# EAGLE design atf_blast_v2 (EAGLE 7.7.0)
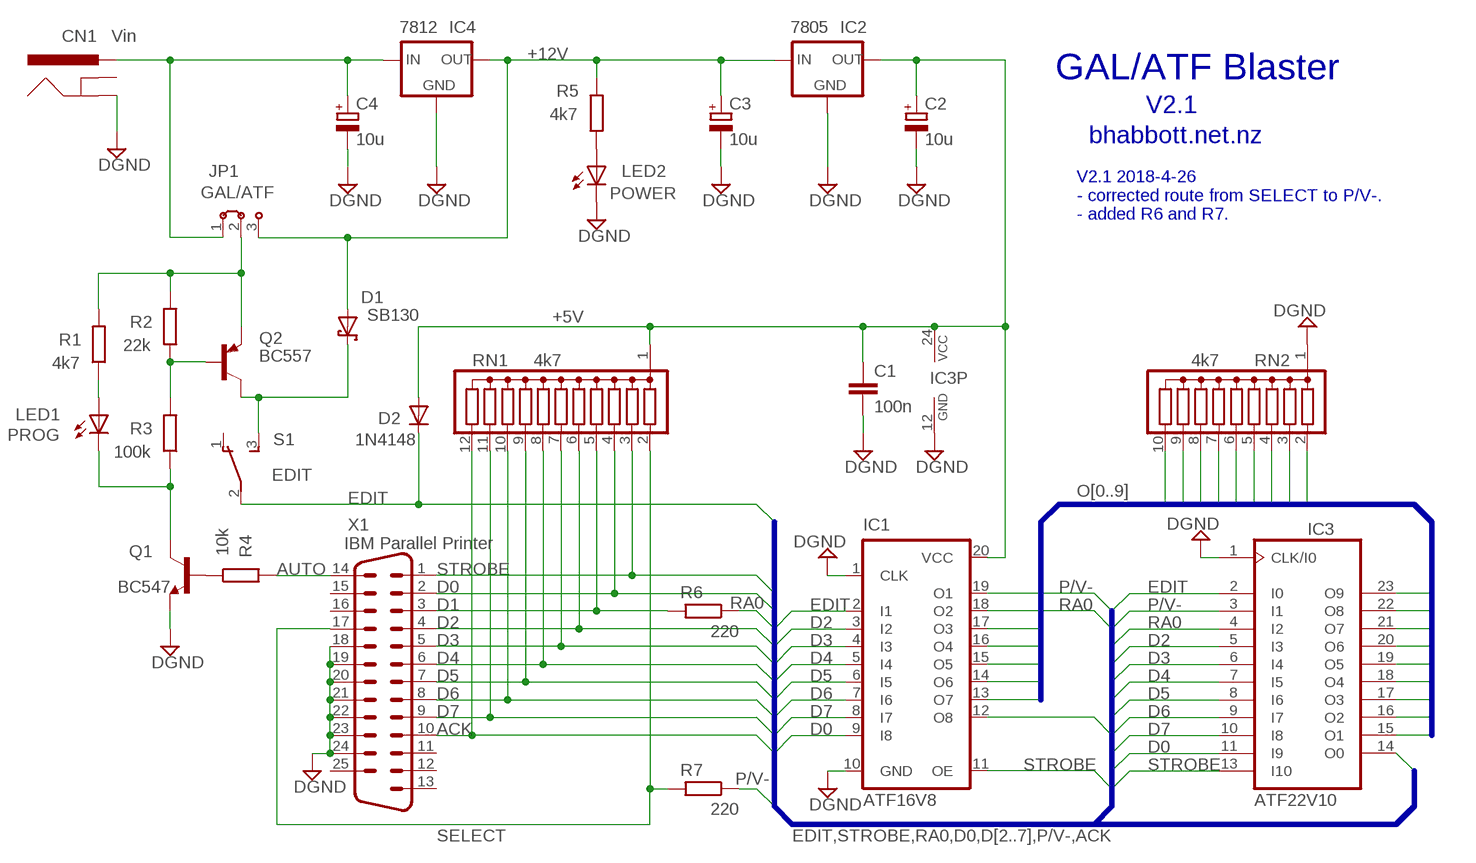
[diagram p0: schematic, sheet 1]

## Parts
C1  100n  C-EU025-024X044  [C025-024X044]
C2  10u  CPOL-EUE2.5-5  [E2,5-5]
C3  10u  CPOL-EUE2.5-5  [E2,5-5]
C4  10u  CPOL-EUE2.5-5  [E2,5-5]
CN1  Vin  POWER_JACKSLT  [POWER_JACK_SLOT]
D1  SB130  SCHOTTKY-DIODEDO35-7  [DO35-7]
D2  1N4148  1N4148DO35-7  [DO35-7]
IC1  ATF16V8  ATF16V8BP3  [DIL20]
IC2  7805  78XXLNV  [78XXL_GND]
IC3  ATF22V10  22V10  [DIL24-3]
IC4  7812  78XXLNV  [78XXL_GND]
JP1  GAL/ATF  JP2N  [0256]
LED1  PROG  LED5MM  [LED5MM]
LED2  POWER  LED5MM  [LED5MM]
Q1  BC547  [TO92]
Q2  BC557  [TO92]
R1  4k7  R-EU_0204/7  [0204/7]
R2  22k  R-EU_0204/7  [0204/7]
R3  100k  R-EU_0204/7  [0204/7]
R4  10k  R-EU_0204/7  [0204/7]
R5  4k7  R-EU_0204/7  [0204/7]
R6  220  R-EU_0204/7  [0204/7]
R7  220  R-EU_0204/7  [0204/7]
RN1  4k7  G11R  [SIL12]
RN2  4k7  G09R  [SIL10]
S1  EDIT  TL36PO  [TL3XPO]
X1  IBM Parallel Printer  M25HP  [M25HP]

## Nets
+5V: C1.1 C2.+ D2.A IC1.20(VCC) IC2.OUT IC3.24(VCC) RN1.1
+12V: C3.+ D1.A IC2.IN IC4.OUT JP1.3 R5.2
ACK: IC1.12(O8) IC3.14(O0) RN1.12 X1.10
AUTO: R4.2 X1.14
CN1: C4.+ CN1.PWR IC4.IN JP1.1
D0: IC1.9(I8) IC3.11(I9) RN1.4 X1.2
D1: R6.2 RN1.5 X1.3
D2: IC1.3(I2) IC3.5(I3) RN1.6 X1.4
D3: IC1.4(I3) IC3.6(I4) RN1.7 X1.5
D4: IC1.5(I4) IC3.7(I5) RN1.8 X1.6
D5: IC1.6(I5) IC3.8(I6) RN1.9 X1.7
D6: IC1.7(I6) IC3.9(I7) RN1.10 X1.8
D7: IC1.8(I7) IC3.10(I8) RN1.11 X1.9
DGND: C1.2 C2.- C3.- C4.- CN1.GND@2(GND) IC1.1(CLK) IC1.10(GND) IC2.GND IC3.1(CLK/I0) IC3.12(GND) IC4.GND LED2.K(C) Q1.1(E) RN2.1 X1.18 X1.19 X1.20 X1.21 X1.22 X1.23 X1.24
EDIT: D2.C IC1.2(I1) IC3.2(I0) S1.2(P)
N$1: D1.C Q2.3(C) S1.3(S)
N$2: Q2.2(B) R2.1 R3.2
N$3: LED1.K(C) Q1.3(C) R3.1
N$4: Q1.2(B) R4.1
N$6: LED1.A R1.1
N$7: JP1.2 Q2.1(E) R1.2 R2.2
N$22: LED2.A R5.1
O1: IC1.13(O7) IC3.15(O1) RN2.2
O2: IC1.14(O6) IC3.16(O2) RN2.3
O3: IC1.15(O5) IC3.17(O3) RN2.4
O4: IC1.16(O4) IC3.18(O4) RN2.5
O5: IC1.17(O3) IC3.19(O5) RN2.6
O6: IC3.20(O6) RN2.7
O7: IC3.21(O7) RN2.8
O8: IC3.22(O8) RN2.9
O9: IC3.23(O9) RN2.10
P/V-: IC1.19(O1) IC3.3(I1) R7.1
RA0: IC1.18(O2) IC3.4(I2) R6.1
SELECT: R7.2 RN1.2 X1.17
STROBE: IC1.11(OE) IC3.13(I10) RN1.3 X1.1
Unconnected: CN1.GND@1(GNDBREAK) S1.1(O) X1.11 X1.12 X1.13 X1.15 X1.16 X1.25 X1.G1 X1.G2

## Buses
EDIT,STROBE,RA0,D0,D[2..7],P/V-,ACK
O[0..9]

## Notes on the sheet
- GAL/ATF Blaster
- V2.1
- bhabbott.net.nz
- V2.1 2018-4-26 
  - corrected route from SELECT to P/V-. 
  - added R6 and R7.

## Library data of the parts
C1 = rcl:C-EU: CAPACITOR, European symbol
C2-C4 = rcl:CPOL-EU: POLARIZED CAPACITOR, European symbol
CN1 = SparkFun-Connectors:POWER_JACK: Power Jack This is the standard 5.5mm barrel jack for power. The PTH is the most common, proven, reliable, footprint. The Slot footprint only works if the mill layer is transmitted to the PCB fab house so be warned. Mating wall wart : TOL-00298 (and others); PROD_ID: PRT-00119
D1 = diode:SCHOTTKY-DIODE: Schottky Diode
D2 = diode:1N4148: DIODE
IC1 = atmel:ATF16V8B: High perfomance CMOS (electrically erasable) programmable logic device (PLD) ABLE-Atmel-ABEL - P18V8R, P16V8C, P16V8AS, P17V8 COPL Atmel-WinCUPL - G16V8MS, G16V8MA, G16V8AS, G16V8 LOG/IC - GAL16V8_R, GAL16V8_G7, GAL16V8_C), GAL16V8 Tango-PLD - G16V8R, G16V8C, G16V8AS, G16V8 Source: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; MPN: ATF16V8CZ-15PU; OC_FARNELL: 1551768; OC_NEWARK: 94M6254
IC2 IC4 = v-reg:78XXL: VOLTAGE REGULATOR
IC3 = pal:22V10: PAL; MPN: GAL22V10D-7LPN; OC_FARNELL: 1571925; OC_NEWARK: 97M0480
JP1 = jumper:JP2N: JUMPER 3 pin 0.1 inch
LED1 LED2 = led:LED: LED
Q1 = transistor-npn:BC547*: NPN Transistor
Q2 = transistor-pnp:BC557: PNP Transistor
R1-R7 = rcl:R-EU_: RESISTOR, European symbol
RN1 = resistor-sil:G11R: SIL RESISTOR; OC_FARNELL: unknown; OC_NEWARK: unknown
RN2 = resistor-sil:G09R: SIL RESISTOR
S1 = switch:TL36PO: TINY SWITCH ON - ON Source: http://www2.produktinfo.conrad.com/datenblaetter/700000-724999/705152-da-01-de-Subminiaturschalter_TL_36YO.pdf
X1 = con-subd:M25HP: SUB-D; OC_FARNELL: unknown; OC_NEWARK: unknown

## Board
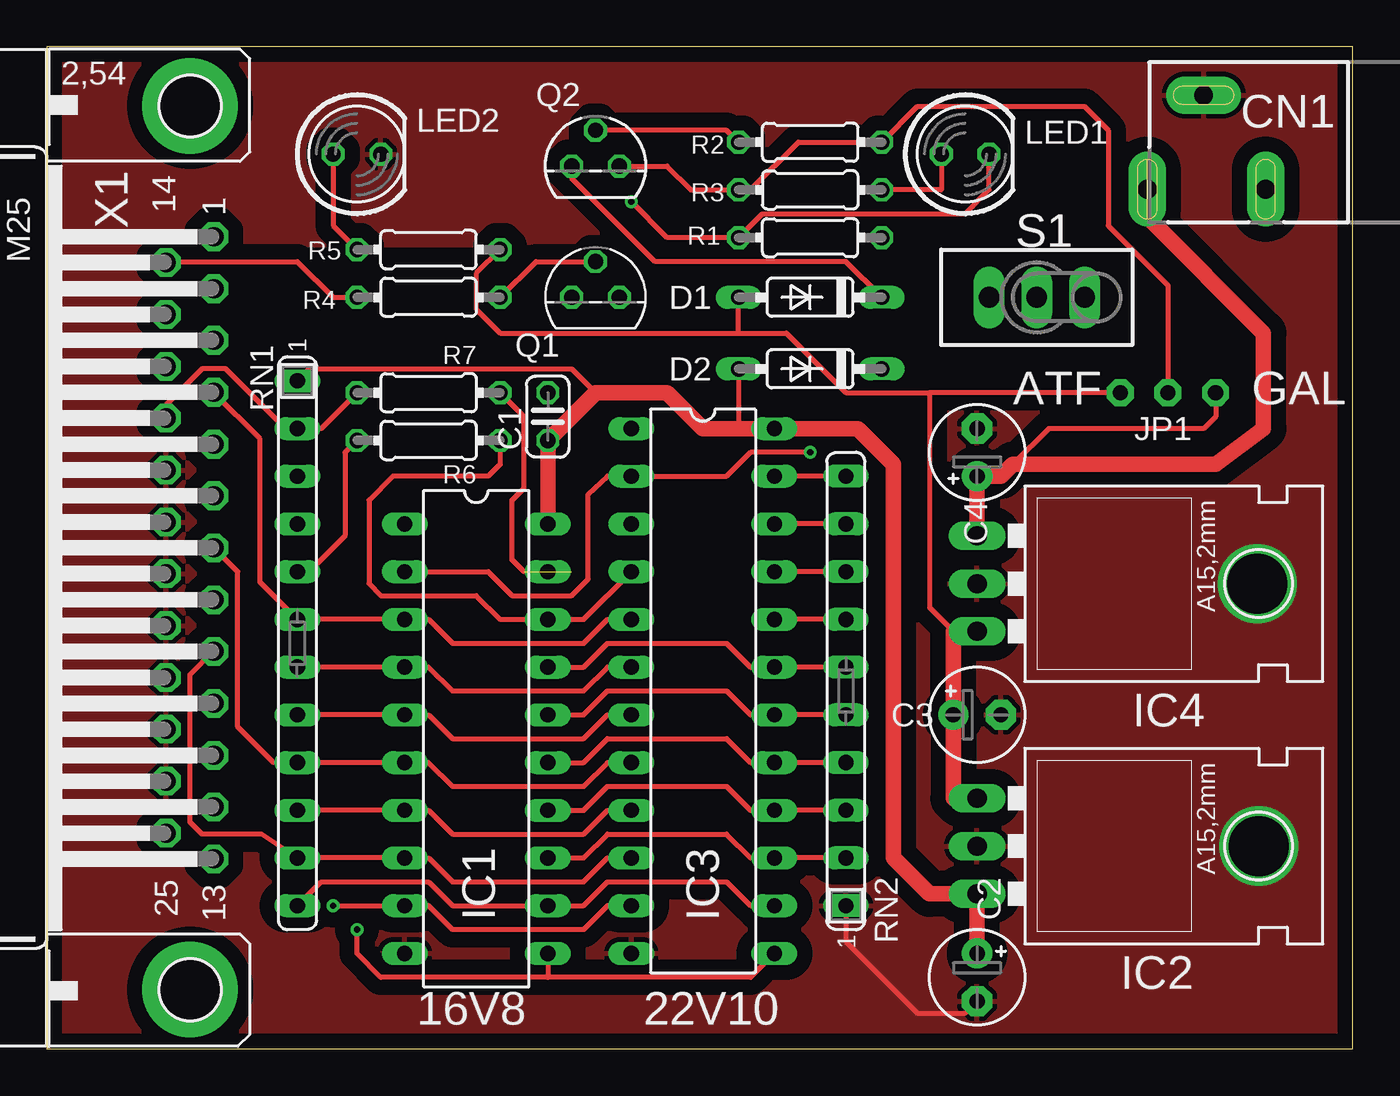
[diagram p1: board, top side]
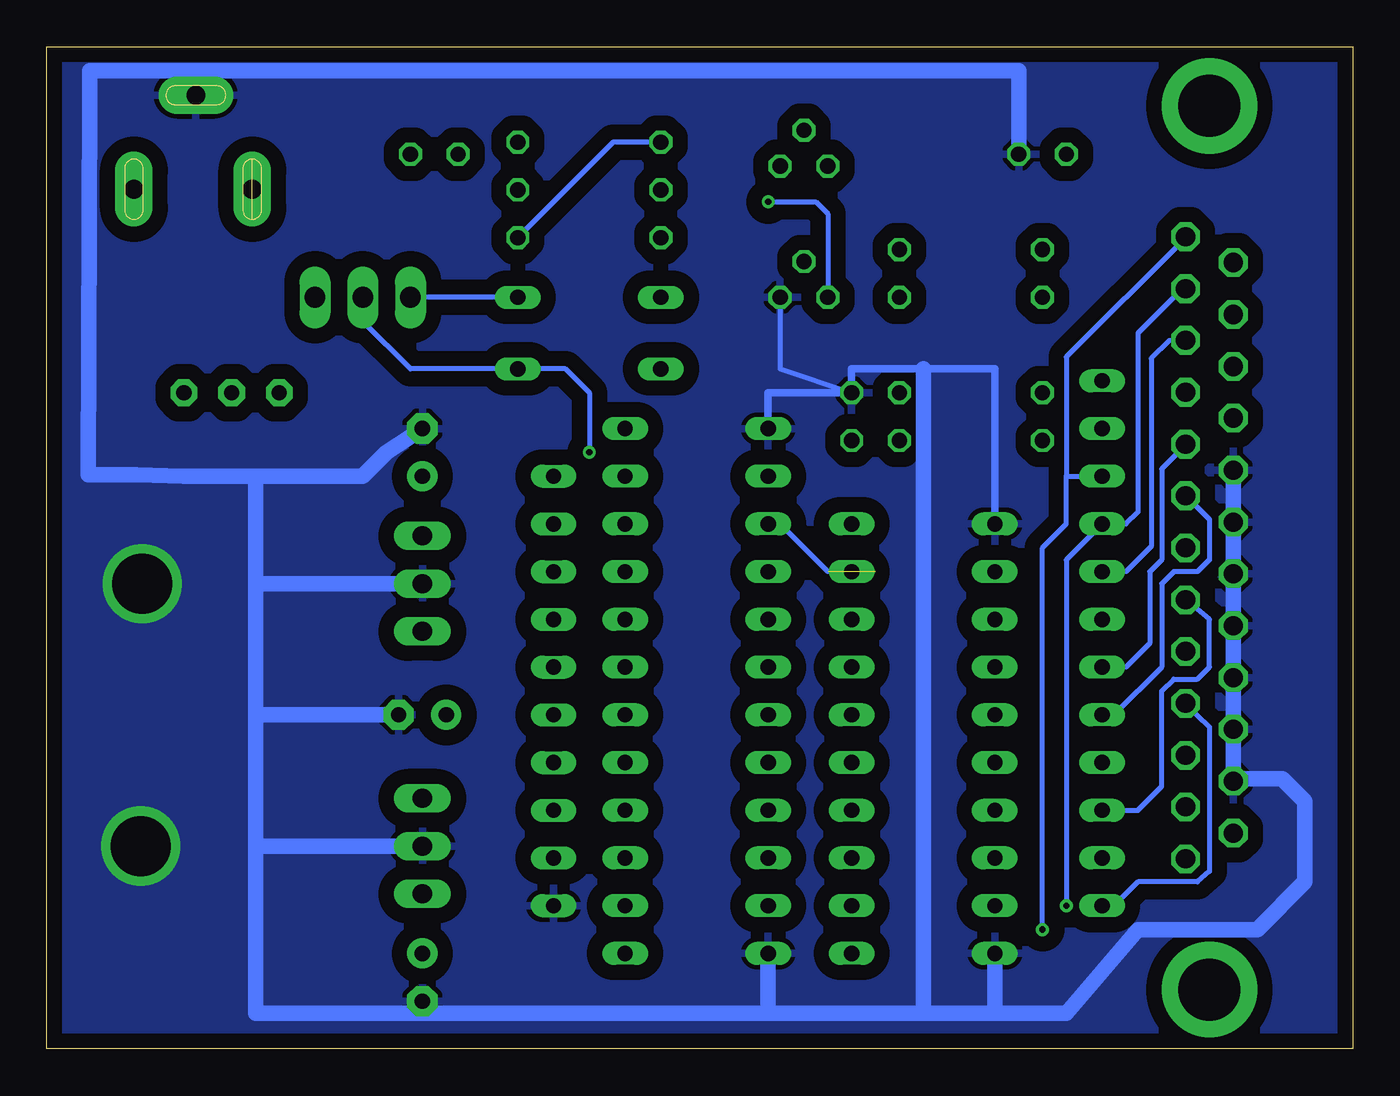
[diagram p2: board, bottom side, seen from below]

Size 69.52 x 53.33 mm. Coordinates in mm from the lower left corner, seen from the top.
Outline: 0,0 69.52,0 69.52,53.33 0,53.33 0,0
Copper layers (1*16): Top 0.0356mm / dielectric 1.5011mm / Bottom 0.0356mm
Design rules "oshpark-10mm": minimum track width 10mil, minimum drill 13mil, track to track 8mil, track to pad 8mil, pad to pad 8mil, via to via 8mil, smd to smd 8mil, copper to edge 15mil, drill to drill 6mil, minimum pad ring 7mil, minimum via ring 7mil, stop-mask expansion 4mil, vias tented up to drill 0mil, thermal gap 10mil

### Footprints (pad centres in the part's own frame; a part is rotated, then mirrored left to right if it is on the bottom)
C025-024X044 = drill 0.813 octagon: 1 -1.27,0; 2 1.27,0
E2,5-5 = drill 0.813 pad 1.6: + -1.27,0 | drill 0.813 pad 1.6 octagon: - 1.27,0
POWER_JACK_SLOT = drill 1 pad 2 long: GND@1 2.58,7.5; GND@2 7.58,10.8; PWR 2.58,13.8
DO35-7 = drill 0.813 long: A 3.81,0; C -3.81,0
DIL20 = drill 0.813 long: 1 -11.43,-3.81; 2 -8.89,-3.81; 3 -6.35,-3.81; 4 -3.81,-3.81; 5 -1.27,-3.81; 6 1.27,-3.81; 7 3.81,-3.81; 8 6.35,-3.81; 9 8.89,-3.81; 10 11.43,-3.81; 11 11.43,3.81; 12 8.89,3.81; 13 6.35,3.81; 14 3.81,3.81; 15 1.27,3.81; 16 -1.27,3.81; 17 -3.81,3.81; 18 -6.35,3.81; 19 -8.89,3.81; 20 -11.43,3.81
78XXL_GND = drill 1.016 long: GND 0,-7.62; IN -2.54,-7.62; OUT 2.54,-7.62
DIL24-3 = drill 0.813 long: 1 -13.97,-3.81; 2 -11.43,-3.81; 3 -8.89,-3.81; 4 -6.35,-3.81; 5 -3.81,-3.81; 6 -1.27,-3.81; 7 1.27,-3.81; 8 3.81,-3.81; 9 6.35,-3.81; 10 8.89,-3.81; 11 11.43,-3.81; 12 13.97,-3.81; 13 13.97,3.81; 14 11.43,3.81; 15 8.89,3.81; 16 6.35,3.81; 17 3.81,3.81; 18 1.27,3.81; 19 -1.27,3.81; 20 -3.81,3.81; 21 -6.35,3.81; 22 -8.89,3.81; 23 -11.43,3.81; 24 -13.97,3.81
0256 = drill 0.813 pad 1.422 octagon: 1 -2.54,0; 2 0,0; 3 2.54,0
LED5MM = drill 0.813 octagon: A -1.27,0; K 1.27,0
TO92 = drill 0.813 octagon: 1 1.27,0; 2 0,1.905; 3 -1.27,0
0204/7 = drill 0.813 octagon: 1 -3.81,0; 2 3.81,0
SIL12 = drill 0.813 long: 1 -13.97,0; 2 -11.43,0; 3 -8.89,0; 4 -6.35,0; 5 -3.81,0; 6 -1.27,0; 7 1.27,0; 8 3.81,0; 9 6.35,0; 10 8.89,0; 11 11.43,0; 12 13.97,0
SIL10 = drill 0.813 long: 1 -11.43,0; 2 -8.89,0; 3 -6.35,0; 4 -3.81,0; 5 -1.27,0; 6 1.27,0; 7 3.81,0; 8 6.35,0; 9 8.89,0; 10 11.43,0
TL3XPO = drill 1.1 pad 1.422 long: 1 -2.54,0; 2 0,0; 3 2.54,0
M25HP = drill 1.016 octagon: 1 -16.561,1.27; 2 -13.792,1.27; 3 -11.049,1.27; 4 -8.28,1.27; 5 -5.512,1.27; 6 -2.769,1.27; 7 0,1.27; 8 2.769,1.27; 9 5.512,1.27; 10 8.28,1.27; 11 11.049,1.27; 12 13.792,1.27; 13 16.561,1.27; 14 -15.189,-1.27; 15 -12.421,-1.27; 16 -9.652,-1.27; 17 -6.909,-1.27; 18 -4.14,-1.27; 19 -1.372,-1.27; 20 1.372,-1.27; 21 4.14,-1.27; 22 6.909,-1.27; 23 9.652,-1.27; 24 12.421,-1.27; 25 15.189,-1.27 | drill 3.302 pad 5.08: G1 -23.52,0; G2 23.52,0

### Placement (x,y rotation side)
C1  26.67,33.66 90 top
C2  49.53,3.81 270 top
C3  49.53,17.78 0 top
C4  49.53,31.75 90 top
CN1  72.39,43.18 90 top
D1  40.64,40.01 180 top
D2  40.64,36.2 180 top
IC1  22.86,16.51 270 top
IC2  57.15,10.79 270 top
IC3  34.92,19.05 270 top
IC4  57.15,24.77 270 top
JP1  59.69,34.92 180 top
LED1  48.9,47.62 0 top
LED2  16.51,47.62 0 top
Q1  29.21,40.01 0 top
Q2  29.21,46.99 0 top
R1  40.64,45.72 180 top
R2  40.64,48.26 0 top
R3  40.64,43.18 0 top
R4  20.32,40.01 180 top
R5  20.32,42.55 0 top
R6  20.32,32.38 180 top
R7  20.32,34.92 180 top
RN1  13.34,21.59 270 top
RN2  42.55,19.05 90 top
S1  52.7,40.01 180 top
X1  7.62,26.67 270 top

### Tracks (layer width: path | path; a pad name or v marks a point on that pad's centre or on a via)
+5V
  Top 0.254: RN1.1 13.97,36.2 27.94,36.2 29.21,34.92 | D2.A 36.83,33.02
  Top 0.813: C2.+ IC2.OUT 46.99,8.26 45.09,10.16 45.09,31.11 43.18,33.02 IC3.24 36.83,33.02 34.92,33.02 33.02,34.92 29.21,34.92 C1.1 IC1.20
+12V
  Top 0.254: R5.2 22.86,41.27 22.86,39.37 24.13,38.1 36.83,38.1 | 36.83,38.1 D1.A | 36.83,38.1 39.37,38.1 42.55,34.92 46.99,34.92 | 46.99,34.92 46.99,23.5 48.26,22.23 | JP1.3 46.99,34.92
  Top 0.813: IC2.IN 48.26,13.34 C3.+ 48.26,22.23 IC4.OUT
ACK
  Top 0.254: RN1.12 14.61,8.89 20.32,8.89 21.59,7.62 IC1.12 28.57,7.62 29.84,8.89 36.2,8.89 37.47,7.62 IC3.14
  Bottom 0.254: RN1.12 12.7,7.62 11.43,8.89 8.26,8.89 7.62,9.45 7.62,17.14 8.89,18.34 X1.10
AUTO
  Top 0.254: R4.2 15.24,40.01 13.34,41.91 6.35,41.91 X1.14
CN1
  Top 0.254: JP1.1 62.23,33.66 61.59,33.02 53.34,33.02 51.44,31.11
  Top 0.813: IC4.IN C4.+ 50.8,30.48 51.44,31.11 62.23,31.11 64.77,33.02 64.77,38.1 58.69,44.18 58.69,46.09 CN1.PWR
D0  (via drill 0.33)
  Top 0.254: IC3.11 29.84,7.62 28.57,6.35 21.59,6.35 20.32,7.62 IC1.9 v15.24,7.62
  Bottom 0.254: X1.2 8.89,40.4 8.97,40.56 11.43,38.1 11.43,28.57 12.06,27.94 RN1.4 15.24,26.04 v15.24,7.62
D1
  Top 0.254: R6.2 15.88,31.75 15.88,27.3 13.97,25.4 RN1.5
  Bottom 0.254: X1.3 9.51,37.72 9.76,37.7 10.72,36.75 10.72,26.75 12.06,25.4 RN1.5
D2
  Top 0.254: IC3.5 29.84,22.86 28.57,21.59 21.59,21.59 20.32,22.86 IC1.3 RN1.6 11.35,24.84 11.35,32.46 8.89,34.92 X1.4
D3
  Top 0.254: RN1.7 IC1.4 20.32,20.32 21.59,19.05 28.57,19.05 29.84,20.32 IC3.6
  Bottom 0.254: X1.5 8.89,32.15 10.16,30.88 10.16,26.04 10.79,25.4 10.79,21.59 12.06,20.32 RN1.7
D4
  Top 0.254: RN1.8 IC1.5 20.32,17.78 21.59,16.51 28.57,16.51 29.84,17.78 IC3.7
  Bottom 0.254: X1.6 7.62,28.18 7.62,26.04 8.26,25.4 9.53,25.4 10.16,24.77 10.16,20.32 12.7,17.78 RN1.8
D5
  Top 0.254: IC3.8 29.84,15.24 28.57,13.97 21.59,13.97 20.32,15.24 IC1.6 RN1.9 12.06,15.24 10.16,17.14 10.16,25.4 X1.7
D6
  Top 0.254: RN1.10 IC1.7 20.32,12.7 21.59,11.43 28.57,11.43 29.84,12.7 IC3.9
  Bottom 0.254: RN1.10 11.43,12.7 10.16,13.97 10.16,19.05 9.53,19.68 8.26,19.68 7.62,20.32 7.62,22.86 X1.8
D7
  Top 0.254: IC3.10 29.84,10.16 28.57,8.89 21.59,8.89 20.32,10.16 IC1.8 RN1.11 11.43,11.43 8.26,11.43 7.62,12.06 7.62,19.92 8.89,21.19 X1.9
DGND  (via drill 3.2)
  Top 0.254: RN2.1 42.55,5.71 46.35,1.91 48.9,1.91 C2.-
  Bottom 0.254: Q1.1 30.48,36.2 C1.2
  Bottom 0.406: X1.24 5.87,14.37 | IC1.1 19.05,36.2 22.86,36.2 26.67,36.2 C1.2 31.11,34.92 IC3.1 | CN1.GND@2
  Bottom 0.813: X1.18 X1.19 X1.20 X1.21 X1.22 X1.23 X1.24 | 5.87,14.37 3.73,14.37 2.54,13.18 2.54,8.89 5.08,6.35 11.43,6.35 15.24,1.91 19.05,1.91 | IC1.10 19.05,1.91 | 19.05,1.91 22.86,1.91 | 22.86,1.91 31.11,1.91 | IC3.12 31.11,1.91 | 31.11,1.91 49.53,1.91 | IC2.GND 58.42,10.79 | 58.42,17.78 58.42,10.79 | 58.42,10.79 58.42,1.91 49.53,1.91 | 49.53,1.91 C2.- | C3.- 58.42,17.78 | 58.42,17.78 58.42,24.77 | 58.42,24.77 58.42,30.48 | 58.42,30.48 62.23,30.48 64.77,30.56 67.31,30.56 67.23,50.72 | 22.86,36.2 22.86,1.91 | 61.59,52.07 17.78,52.07 LED2.K | 61.59,52.07 67.23,52.07 67.23,50.8 | 58.42,30.48 52.7,30.48 51.44,31.75 C4.- | IC4.GND 58.42,24.77 | CN1.GND@2 61.59,52.07
  other vias: 64.45,24.77 64.53,10.79
  pour Bottom (isolate 0.813, rank 6): 0,53.34 69.85,53.34 69.85,0 0,0
  pour Top (isolate 0.813, rank 6): 69.85,53.34 69.85,0 0,0 0,53.34
  cutout Top (isolate 0.813, rank 5): 10.16,42.55 36.2,42.55 36.2,24.13 10.16,24.13
EDIT  (via drill 0.33)
  Top 0.254: v40.64,31.75 37.47,31.75 36.2,30.48 IC3.2 29.84,30.48 28.81,29.53 28.81,25 27.94,24.13 24.77,24.13 23.5,25.4 IC1.2
  Bottom 0.254: v40.64,31.75 40.64,34.92 41.91,36.2 D2.C 50.16,36.2 52.7,38.73 S1.2
N$1
  Top 0.254: Q2.3 27.94,46.35 32.38,41.91 42.55,41.91 D1.C
  Bottom 0.254: D1.C S1.3
N$2
  Top 0.254: Q2.2 36.2,48.9 R2.1
  Bottom 0.254: R3.2 39.37,48.26 R2.1
N$3  (via drill 0.33)
  Top 0.254: v31.11,45.09 33.02,43.18 R3.1 38.1,44.45 48.9,44.45 50.16,45.72 LED1.K
  Bottom 0.254: Q1.3 27.94,44.45 28.57,45.09 v31.11,45.09
N$4
  Top 0.254: R4.1 26.04,41.91 Q1.2
N$6
  Top 0.254: LED1.A 47.62,45.72 R1.1
N$7
  Top 0.254: Q2.1 33.02,46.99 34.29,45.72 R1.2 37.47,45.72 40.01,48.26 R2.2 46.35,50.16 55.24,50.16 56.52,48.9 56.52,43.81 59.69,40.64 JP1.2
N$22
  Top 0.254: LED2.A 15.24,43.81 R5.1
O1
  Top 0.254: IC1.13 28.57,10.16 29.84,11.43 36.2,11.43 37.47,10.16 IC3.15 RN2.2
O2
  Top 0.254: IC1.14 28.57,12.7 29.84,13.97 36.2,13.97 37.47,12.7 IC3.16 RN2.3
O3
  Top 0.254: IC1.15 28.57,15.24 29.84,16.51 36.2,16.51 37.47,15.24 IC3.17 RN2.4
O4
  Top 0.254: IC1.16 28.57,17.78 29.84,19.05 36.2,19.05 37.47,17.78 IC3.18 RN2.5
O5
  Top 0.254: IC1.17 28.57,20.32 29.84,21.59 36.2,21.59 37.47,20.32 IC3.19 RN2.6
O6
  Top 0.254: RN2.7 IC3.20
O7
  Top 0.254: RN2.8 IC3.21
O8
  Top 0.254: RN2.9 IC3.22
O9
  Top 0.254: RN2.10 IC3.23
P/V-  (2 unrouted)
  Top 0.254: 25.4,25.4 24.77,26.04 24.77,29.21 25.4,29.84 25.4,33.66 R7.1
  Bottom 0.254: 27.94,25.4 30.48,27.94 IC3.3
RA0
  Top 0.254: R6.1 24.13,31.11 23.5,30.48 18.41,30.48 17.14,29.21 17.14,24.77 17.78,24.13 22.86,24.13 24.13,22.86 IC1.18 28.57,22.86 IC3.4
SELECT
  Top 0.254: X1.17 6.35,34.29 8.26,36.2 9.53,36.2 12.7,33.02 RN1.2 14.61,33.02 R7.2
STROBE  (via drill 0.33)
  Top 0.254: 26.67,3.81 37.47,3.81 IC3.13 | IC1.11 26.67,3.81 | 26.67,3.81 17.78,3.81 16.51,5.08 v16.51,6.35
  Bottom 0.254: 15.24,30.48 15.24,36.83 8.97,43.1 8.89,43.1 X1.1 8.89,43.26 | v16.51,6.35 16.51,26.67 15.24,27.94 15.24,30.48 | 15.24,30.48 RN1.3

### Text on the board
tNames: ATF | GAL | 16V8 | 22V10

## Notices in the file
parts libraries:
SparkFun-Connectors: Licensing: Creative Commons ShareAlike 4.0 International - https://creativecommons.org/licenses/by-sa/4.0
